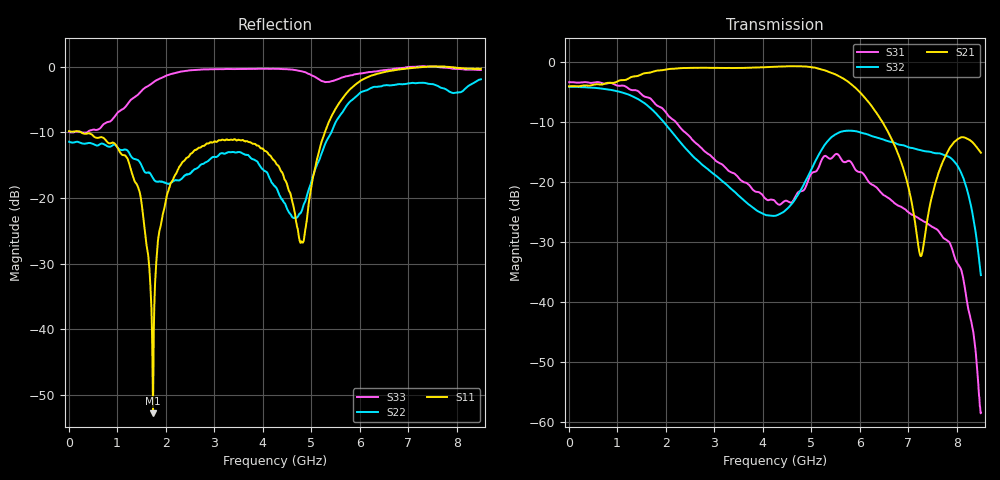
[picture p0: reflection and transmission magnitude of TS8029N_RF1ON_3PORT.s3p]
!Created with skrf (http://scikit-rf.org).
# GHz S RI R 50.0
!freq ReS11 ImS11 ReS12 ImS12 ReS13 ImS13
! ReS21 ImS21 ReS22 ImS22 ReS23 ImS23
! ReS31 ImS31 ReS32 ImS32 ReS33 ImS33
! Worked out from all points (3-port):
!   1601 points, 10 MHz to 8.5 GHz, reference 50 ohm
!   strongest paths, dB at 10 MHz, 2.132 GHz, 4.255 GHz, 6.378 GHz, 8.5 GHz:
!     S21: -4.1, -1.2, -0.9, -8.9, -15.2
!     S32: -4.2, -11.7, -25.6, -12.7, -35.5
!     S31: -3.4, -9.6, -23.2, -21.2, -58.4
!   lowest |S11| = -52.8 dB at 1.74 GHz (marker M1), VSWR 1.00, Z = 50.2 + j0.135 ohm
!   |S11| at or under -10 dB: 253.9 MHz to 5.281 GHz (5.028 GHz wide, 182 % of centre)
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0.01  -0.3223 0.00625  0.6231 0.00125  0.6736 -0.00405
      0.623 0.00122  -0.2675 0.00677  0.6171 -0.00527
      0.6734 -0.00418  0.6172 -0.00519  -0.3181 0.0113
1.219825  -0.1542 0.1229  0.694 -0.1801  0.1561 -0.5824
          0.6942 -0.1804  -0.1573 0.1651  0.0885 -0.5269
          0.1556 -0.5823  0.0885 -0.5272  0.4663 0.2317
1.739837  0.00185 0.00135  0.7249 -0.3938  -0.1614 -0.4393
          0.7246 -0.394  -0.1023 0.098  -0.1984 -0.3378
          -0.161 -0.4393  -0.1984 -0.3381  0.6774 -0.3344
2.318219  0.0785 -0.1622  0.5927 -0.6536  -0.2121 -0.1787
          0.5929 -0.6536  -0.1148 0.0777  -0.1853 -0.098
          -0.2118 -0.179  -0.1856 -0.098  0.4672 -0.7872
4.255  -0.0571 -0.1808  -0.2952 -0.8564  -0.0672 0.0158
       -0.2954 -0.8564  0.0725 0.099  -0.0389 0.0351
       -0.0673 0.016  -0.0388 0.035  -0.4856 -0.8291
4.812156  0.04 -0.0229  -0.6257 -0.665  -0.0659 0.0516
          -0.626 -0.665  0.00559 -0.0806  -0.0265 0.0854
          -0.0661 0.0517  -0.0263 0.0851  -0.8075 -0.438
5.332169  0.31 0.168  -0.7922 -0.2509  0.091 0.1325
          -0.7927 -0.2506  -0.2775 -0.0198  0.1471 0.1584
          0.0911 0.1324  0.1469 0.1581  0.00797 0.7638
6.536688  0.8574 -0.314  -0.1785 0.2188  -0.013 -0.0748
          -0.1781 0.2184  0.0166 0.7204  0.0677 -0.2097
          -0.0131 -0.0747  0.0676 -0.2102  0.5228 -0.782
7.513038  0.8823 -0.477  -0.0428 -0.0706  -0.0336 -0.025
          -0.0424 -0.0706  0.7338 -0.022  -0.0842 -0.1528
          -0.0335 -0.0252  -0.0851 -0.1525  0.5335 -0.8466
8.5  0.7006 -0.6586  -0.16 0.0689  0.000985 0.000743
     -0.1604 0.0692  -0.7935 0.0999  -0.015 -0.00784
     0.000932 0.000761  -0.0149 -0.00772  0.3171 -0.8874
